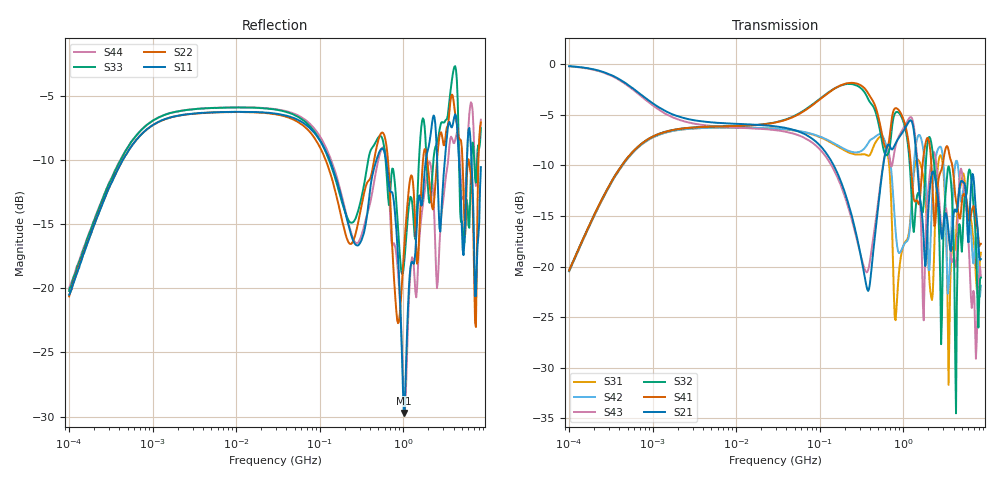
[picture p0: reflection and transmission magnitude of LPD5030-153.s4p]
# MHz S MA R 50
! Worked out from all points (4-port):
!   498 points, 100 kHz to 8.5 GHz, reference 50 ohm
!   strongest paths, dB at 100 kHz, 1.698 MHz, 29.49 MHz, 500.7 MHz, 8.5 GHz:
!     S21: -0.2, -4.9, -6.1, -14.1, -19.3
!     S41: -20.4, -6.5, -5.8, -5.1, -17.7
!     S32: -20.4, -6.5, -5.7, -5.7, -21.1
!     S43: -0.2, -5.2, -6.5, -13.6, -21.0
!     S42: -20.5, -6.6, -6.4, -7.0, -21.9
!     S31: -20.5, -6.6, -6.4, -7.3, -18.6
!   lowest |S11| = -29.7 dB at 1.016 GHz (marker M1), VSWR 1.07, Z = 47.1 - j1.33 ohm
!   |S11| at or under -10 dB: 620.5 MHz to 1.867 GHz (1.247 GHz wide, 100 % of centre); 4.651 GHz to 5.79 GHz (1.14 GHz wide, 21.8 % of centre); 6.558 GHz to end of sweep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
0.1  0.09439 76.5  0.9772 -5.4  0.09495 -101.6  0.09553 78.4
     0.9772 -5.4  0.09295 76.5  0.09519 78.4  0.09467 -101.7
     0.09495 -101.6  0.09519 78.4  0.09762 75.5  0.9751 -5.7
     0.09553 78.4  0.09467 -101.7  0.9751 -5.7  0.09918 76.5
167.2873  0.25 -59.8  0.2824 -90.7  0.39 80.2  0.776 -19.4
          0.2824 -90.7  0.2128 -57.3  0.7754 -22.4  0.3955 76.6
          0.39 80.2  0.7754 -22.4  0.2426 -50.7  0.2691 -93.7
          0.776 -19.4  0.3955 76.6  0.2691 -93.7  0.2574 -63.9
601.0223  0.3344 -105.3  0.3529 24.7  0.4142 -82.2  0.3927 -105.9
          0.3529 24.7  0.3887 -108.1  0.3619 -111.1  0.4168 -74.6
          0.4142 -82.2  0.3619 -111.1  0.3394 -102.8  0.3553 21.0
          0.3927 -105.9  0.4168 -74.6  0.3553 21.0  0.3478 -116.8
1016.278  0.03271 -154.4  0.471 -101.5  0.1282 -100.1  0.5272 -173.4
          0.471 -101.5  0.1375 -101.3  0.5114 177.6  0.128 -111.0
          0.1282 -100.1  0.5114 177.6  0.1219 -125.0  0.4864 -99.9
          0.5272 -173.4  0.128 -111.0  0.4864 -99.9  0.03672 -172.7
2905.739  0.2177 8.6  0.1371 -18.1  0.342 -36.4  0.3071 -15.6
          0.1371 -18.1  0.3947 -0.3  0.05589 -4.5  0.3743 -46.0
          0.342 -36.4  0.05589 -4.5  0.4435 -5.5  0.1485 -34.1
          0.3071 -15.6  0.3743 -46.0  0.1485 -34.1  0.202 28.0
4187.455  0.4756 -157.3  0.1914 -155.0  0.1223 -153.7  0.2259 143.0
          0.1914 -155.0  0.477 -168.2  0.03618 64.7  0.3184 -175.0
          0.1223 -153.7  0.03618 64.7  0.7321 -175.1  0.09962 -167.0
          0.2259 143.0  0.3184 -175.0  0.09962 -167.0  0.3771 -141.1
8500  0.2962 -25.9  0.1089 -8.2  0.117 -20.7  0.1296 -34.6
      0.1089 -8.2  0.442 -47.6  0.08822 34.8  0.0804 -10.3
      0.117 -20.7  0.08822 34.8  0.42 -31.1  0.08887 5.6
      0.1296 -34.6  0.0804 -10.3  0.08887 5.6  0.4531 -29.8
